(* Logix 5000 AddOnInstructionDefinition export HI1769_AOI_INT; software revision 32.00 *)

TYPE HardyCmdResult :   // Results returned for commands without specific data associated with command.
STRUCT
   Cmd : INT;
   CmdStatus : INT;
END_STRUCT
END_TYPE

TYPE HardyIntParam0 :   // parameter 0 values using integer values.
STRUCT
   ChanActive : INT;
   Metric : INT;
   Waversaver : INT;
   NumAverages : INT;
   ZeroTrackEnable : INT;
   ROC_Time_Base : INT;
   AutoZeroTol : DINT;
   MotionTol : DINT;
   ZeroTol : DINT;
   unused1 : INT;
   unused2 : INT;
END_STRUCT
END_TYPE

TYPE HardyIntParam1 :   // parameter 1 values with integer variables.
STRUCT
   TareWeight : DINT;
   SpanWeight : DINT;
   CalLowWeight : DINT;
   ZeroCount : DINT;
   CalZeroCount : DINT;
   CalLowCount : DINT;
   CalHighCount : DINT;
END_STRUCT
END_TYPE

TYPE HardyIntWeight :   // default return from module when no command given.
STRUCT
   Channel_Status : INT;
   FirmwareRev : INT;
   Gross_Weight : DINT;
   Net_Weight : DINT;
   Metric : INT;
   CalType : INT;
   ADC_Counts : DINT;
   Rate_of_Change : DINT;
   Serial_Number : INT;
   Conv_Count : INT;
END_STRUCT
END_TYPE

ADD_ON_INSTRUCTION HI1769_AOI_INT   (* revision 1.0 *)
// To operate with a single channel of an HI 1769 WS or HI 1769-2WS module.
// Revision note:
// Complete rewrite of the AOI to operate with a single channel of a module even if it is a two channel module.  This allows the user to set up each channel in the format they wish without regard to the way the other channel is configured.
VAR_IN_OUT
   Inp_hi1769 : HI:1769_xWS_ChannelNOCMD_r3:I:0; {required}
   Out_hi1769 : HI:1769_xWS_Channel:O:0; {required}
END_VAR
VAR_INPUT
   auto_zero_flt : REAL;   // auto zero tolerance float format
   auto_zero_int : DINT;   // auto zero tolerance integer format
   C2_cal_cmd : BOOL;   // trigger the C2 cal command
   cal_hi_cmd : BOOL;   // trigger the cal high command
   cal_low_cmd : BOOL;   // trigger the cal low command
   callow_wt_flt : REAL;   // Cal low reference weight float format
   callow_wt_int : DINT;   // Cal low reference weight integer format
   capacity : REAL;   // capacity of scale
   chan_enable : INT;   // Channel enabled indication
   chan_status : INT;   // channel status
   decimal_pt : INT;   // decimal point positions if integer format module
   metric : INT;   // Metric setting for units, format, decimal
   mot_tol_flt : REAL;   // motion tolerance float format
   mot_tol_int : DINT;   // motion tolerance integer format
   num_avg : INT;   // Averages
   rd_param_0_1 : BOOL;   // trigger read param 0 data from page 1 of configuration
   rd_param_0_2 : BOOL;   // trigger read param 0 data from page 2 of configuration
   rd_param_1_c2 : BOOL;   // trigger read param 1 data from C2 cal page
   rd_param_1_trad : BOOL;   // trigger read param 1 data from traditional cal page
   roc_tb : INT;   // ROC time base
   save_params0 : BOOL;   // trigger write of configuration parameters
   save_params0_2 : BOOL;   // trigger write of param0 config data from page 2 of config
   save_params1 : BOOL;   // trigger write of param 1 from C2 cal page
   save_params1_1 : BOOL;   // triggers save of cal parameters from traditional cal page
   Set_FaceplateAnimation : INT;   // sets the page of display on HMI
   span_wt_flt : REAL;   // Span ref weight float format
   span_wt_int : DINT;   // span ref weight integer format
   tare_cmd : BOOL;   // triggers tare command
   tare_wt_flt : REAL;   // tare weight float format
   tare_wt_int : DINT;   // tare weight integer format
   unit : INT;   // units of measure
   waversaver : INT;   // WAVERSAVER filter setting
   zero_cmd : BOOL;   // triggers zero command
   zero_tol_flt : REAL;   // zero tolerance float format
   zero_tol_int : DINT;   // zero tolerance integer format
   zero_trk_enable : INT;   // zero track enable
END_VAR
VAR_OUTPUT
   active : BOOL;
   cmd_status : INT;
   current_metric : INT; {access Read Only}   // current metric setting
   fp_dis_md : DINT;   // set display of gross or net weight for HMI
   gross_wt_flt : REAL; {access Read Only}   // Gross weight float format
   gross_wt_int : DINT; {access Read Only}   // gross weight integer format
   ins_status : INT;   // instrument status
   net_wt_flt : REAL; {access Read Only}   // net weight float format
   net_wt_int : DINT; {access Read Only}   // net weight integer format
   percent : REAL; {access Read Only}   // weight in percentage of capacity for gauge
   roc_flt : REAL; {access Read Only}   // Rate of Change in float format
   roc_int : DINT; {access Read Only}   // Rate of Change in integer format
END_VAR
VAR
   C2_cal_ctrl : DINT; {access None}
   C2_cmd_reset_timer : TIMER := (PRE := 3000); {access None}
   cal_data_xfer_delay : TIMER := (PRE := 200); {access None}
   cal_hi_ctrl : DINT; {access None}
   cal_lo_ctrl : DINT; {access None}
   CalHI_cmd_reset_timer : TIMER := (PRE := 3000); {access None}
   CalLo_cmd_reset_timer : TIMER := (PRE := 3000); {access None}
   clr_cmd : BOOL; {access None}
   comm_ck_timer : TIMER := (PRE := 3000); {access None}   // communications check timer
   config_data_xfer_delay_timer : TIMER := (PRE := 200); {access None}
   copy_cal_data_delay : TIMER := (PRE := 200); {access None}
   default_return_int : HardyIntWeight; {access None}
   init_metric : BOOL; {access None}
   init_timer : TIMER := (PRE := 1000); {access None}
   no_update : BOOL; {access None}   // communication loss indication
   one_shot_clr_1 : BOOL; {access None}
   one_shot_clr_2 : BOOL; {access None}
   one_shot_metric : BOOL; {access None}
   previous_count : INT; {access None}
   rd_config_data_delay : TIMER := (PRE := 200); {access None}
   rd_param0_ctrl : DINT; {access None}
   rd_param1_ctrl : DINT; {access None}
   Read_Int_param_0 : HardyIntParam0; {access None}
   Read_Int_param_1 : HardyIntParam1; {access None}
   reset_cmd_delay_timer : TIMER := (PRE := 1000); {access None}
   save_cal_delay_timer : TIMER := (PRE := 200); {access None}
   save_config_delay_timer : TIMER := (PRE := 200); {access None}
   save_param0_delay_timer : TIMER := (PRE := 3000); {access None}
   save_param1_delay_timer : TIMER := (PRE := 3000); {access None}
   start_reset_cmd_delay_timer : BOOL; {access None}   // reset read command delay
   Status_Return : HardyCmdResult; {access None}
   tare_cmd_reset_timer : TIMER := (PRE := 3000); {access None}
   tare_ctrl : DINT; {access None}
   wr_param0_ctrl : DINT; {access None}
   wr_param1_ctrl : DINT; {access None}
   write_int_param_0 : HardyIntParam0; {access None}
   write_int_param_1 : HardyIntParam1; {access None}
   zero_cmd_reset_timer : TIMER := (PRE := 3000); {access None}
   zero_ctrl : DINT; {access None}
END_VAR

ROUTINE Logic   (* ladder *)
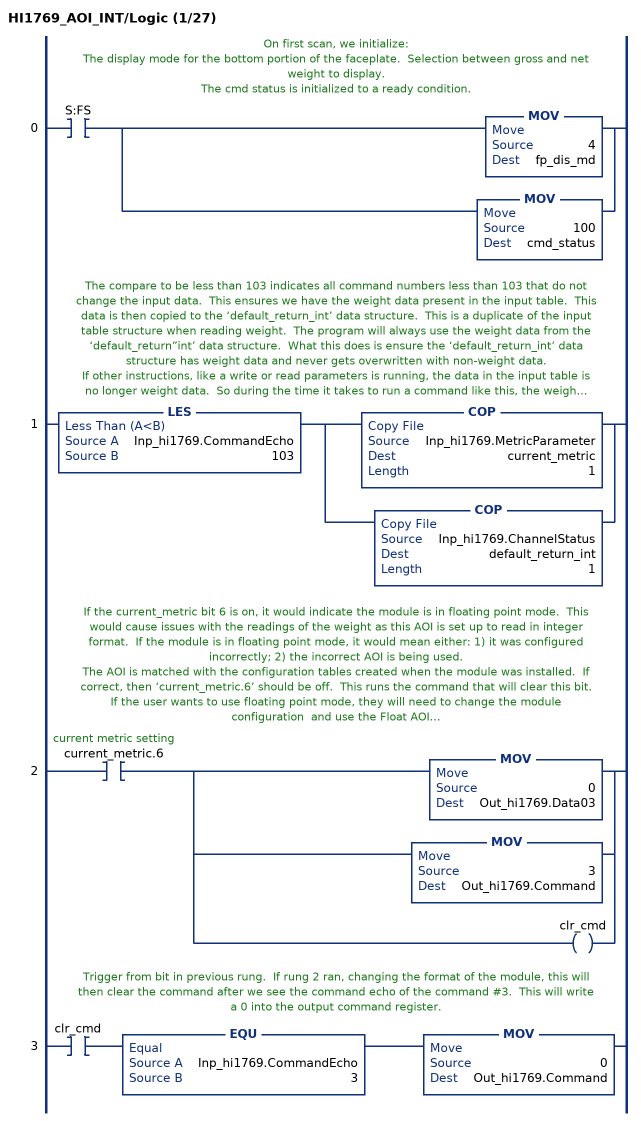
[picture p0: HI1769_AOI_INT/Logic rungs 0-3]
   // On first scan, we initialize:
   // The display mode for the bottom portion of the faceplate.  Selection between gross and net weight to display.
   // The cmd status is initialized to a ready condition.
   0: XIC(S:FS)[MOV(4,fp_dis_md) ,MOV(100,cmd_status) ];
   // The compare to be less than 103 indicates all command numbers less than 103 that do not change the input data.  This ensures we have the weight data present in the input table.  This data is then copied to the ‘default_return_int’ data structure.  This is a duplicate of the input table structure when reading weight.  The program will always use the weight data from the ‘default_return”int’ data structure.  What this does is ensure the ‘default_return_int’ data structure has weight data and never gets overwritten with non-weight data.
   // If other instructions, like a write or read parameters is running, the data in the input table is no longer weight data.  So during the time it takes to run a command like this, the weight data is taken from the ‘default_return_int’ structure instead of the input table.  The weight will not change during this time frame, but it is so short it should not matter.  However, this prevents using values as weight when the values are not weight values.
   // This also copies the metric setting to the ‘current_metric’ tag.  This tag is used to read the: Units of measure and decimal point value.
   1: LES(Inp_hi1769.CommandEcho,103)[COP(Inp_hi1769.MetricParameter,current_metric,1) ,COP(Inp_hi1769.ChannelStatus,default_return_int,1) ];
   // If the current_metric bit 6 is on, it would indicate the module is in floating point mode.  This would cause issues with the readings of the weight as this AOI is set up to read in integer format.  If the module is in floating point mode, it would mean either: 1) it was configured incorrectly; 2) the incorrect AOI is being used.
   // The AOI is matched with the configuration tables created when the module was installed.  If correct, then ‘current_metric.6’ should be off.  This runs the command that will clear this bit.
   // If the user wants to use floating point mode, they will need to change the module configuration  and use the Float AOI.
   // The command #3 writes to the metric setting in the module.  Moving the 0 into Data03 will write a 0 in for the metric setting.  This will turn off the floating point format.
   // If the bit is not set, indicating the module is in Integer format, then this rung will be skipped.
   2: XIC(current_metric.6)[MOV(0,Out_hi1769.Data03) ,MOV(3,Out_hi1769.Command) ,OTE(clr_cmd) ];
   // Trigger from bit in previous rung.  If rung 2 ran, changing the format of the module, this will then clear the command after we see the command echo of the command #3.  This will write a 0 into the output command register.
   3: XIC(clr_cmd)EQU(Inp_hi1769.CommandEcho,3)MOV(0,Out_hi1769.Command);
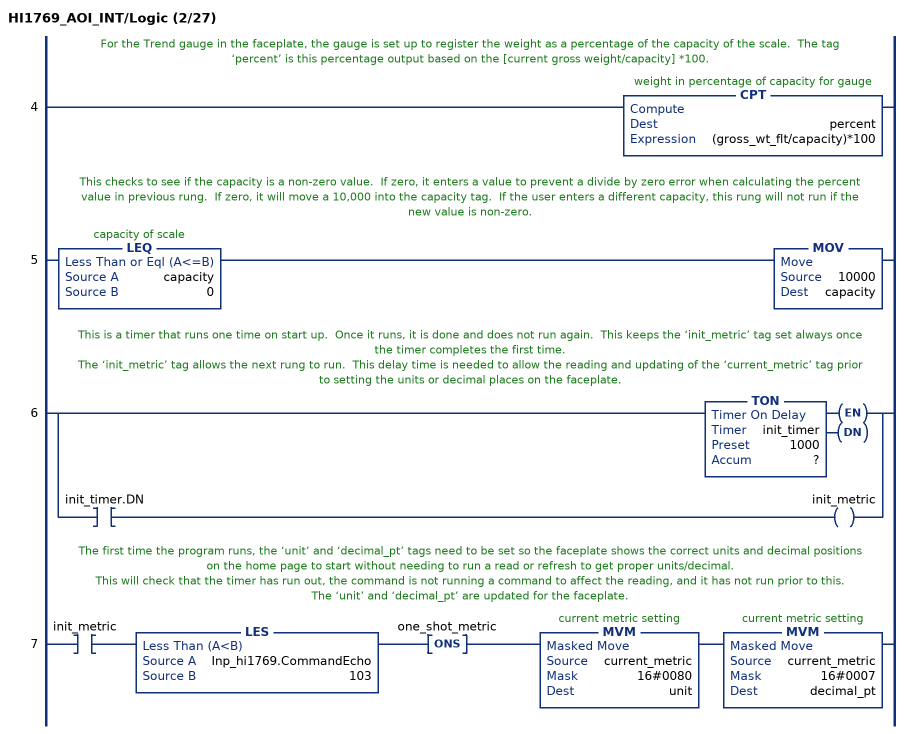
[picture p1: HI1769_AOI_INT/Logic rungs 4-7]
   // For the Trend gauge in the faceplate, the gauge is set up to register the weight as a percentage of the capacity of the scale.  The tag ‘percent’ is this percentage output based on the [current gross weight/capacity] *100.
   4: CPT(percent,(gross_wt_flt/capacity)*100);
   // This checks to see if the capacity is a non-zero value.  If zero, it enters a value to prevent a divide by zero error when calculating the percent value in previous rung.  If zero, it will move a 10,000 into the capacity tag.  If the user enters a different capacity, this rung will not run if the new value is non-zero.
   5: LEQ(capacity,0)MOV(10000,capacity);
   // This is a timer that runs one time on start up.  Once it runs, it is done and does not run again.  This keeps the ‘init_metric’ tag set always once the timer completes the first time.
   // The ‘init_metric’ tag allows the next rung to run.  This delay time is needed to allow the reading and updating of the ‘current_metric’ tag prior to setting the units or decimal places on the faceplate.
   6: [TON(init_timer,?,?) ,XIC(init_timer.DN) OTE(init_metric) ];
   // The first time the program runs, the ‘unit’ and ‘decimal_pt’ tags need to be set so the faceplate shows the correct units and decimal positions on the home page to start without needing to run a read or refresh to get proper units/decimal.
   // This will check that the timer has run out, the command is not running a command to affect the reading, and it has not run prior to this.
   // The ‘unit’ and ‘decimal_pt’ are updated for the faceplate.
   7: XIC(init_metric)LES(Inp_hi1769.CommandEcho,103)ONS(one_shot_metric)MVM(current_metric,16#0080,unit)MVM(current_metric,16#0007,decimal_pt);
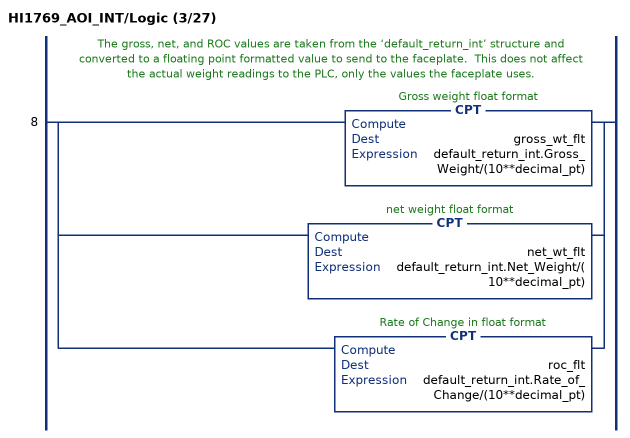
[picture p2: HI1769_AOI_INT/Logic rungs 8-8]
   // The gross, net, and ROC values are taken from the ‘default_return_int’ structure and converted to a floating point formatted value to send to the faceplate.  This does not affect the actual weight readings to the PLC, only the values the faceplate uses.
   8: [CPT(gross_wt_flt,default_return_int.Gross_Weight/(10**decimal_pt)) ,CPT(net_wt_flt,default_return_int.Net_Weight/(10**decimal_pt)) ,CPT(roc_flt,default_return_int.Rate_of_Change/(10**decimal_pt)) ];
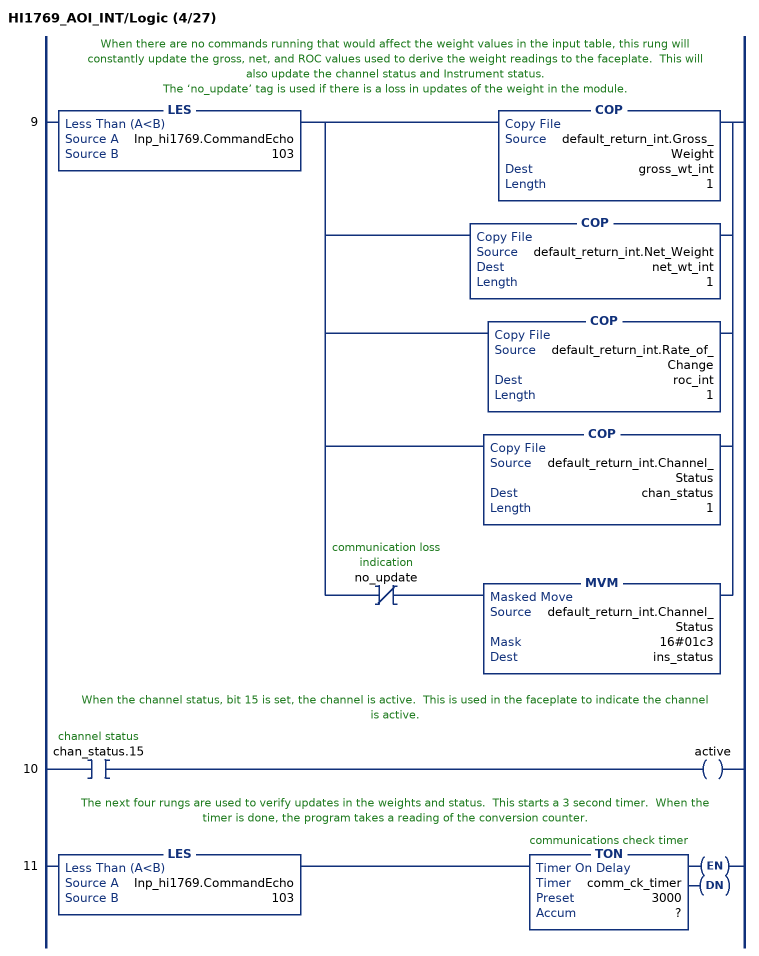
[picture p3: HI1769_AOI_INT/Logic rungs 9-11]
   // When there are no commands running that would affect the weight values in the input table, this rung will constantly update the gross, net, and ROC values used to derive the weight readings to the faceplate.  This will also update the channel status and Instrument status.
   // The ‘no_update’ tag is used if there is a loss in updates of the weight in the module.
   9: LES(Inp_hi1769.CommandEcho,103)[COP(default_return_int.Gross_Weight,gross_wt_int,1) ,COP(default_return_int.Net_Weight,net_wt_int,1) ,COP(default_return_int.Rate_of_Change,roc_int,1) ,COP(default_return_int.Channel_Status,chan_status,1) ,XIO(no_update) MVM(default_return_int.Channel_Status,16#01c3,ins_status) ];
   // When the channel status, bit 15 is set, the channel is active.  This is used in the faceplate to indicate the channel is active.
   10: XIC(chan_status.15)OTE(active);
   // The next four rungs are used to verify updates in the weights and status.  This starts a 3 second timer.  When the timer is done, the program takes a reading of the conversion counter.
   11: LES(Inp_hi1769.CommandEcho,103)TON(comm_ck_timer,?,?);
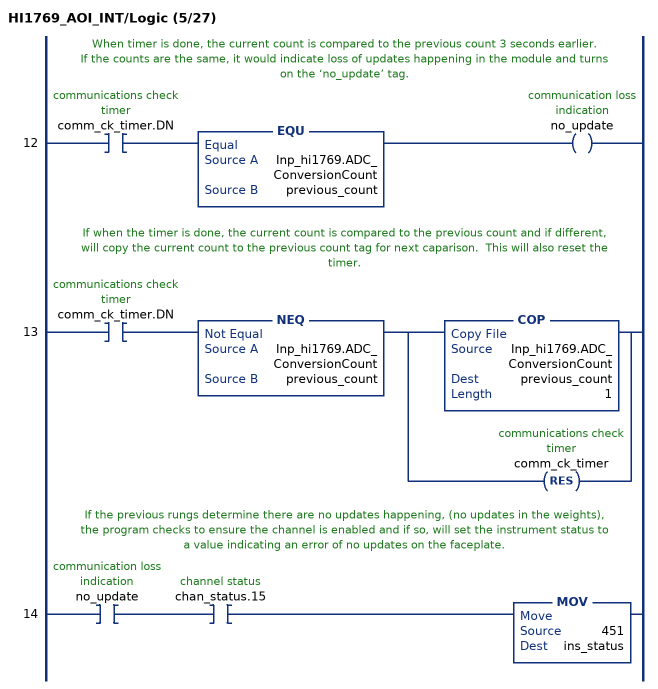
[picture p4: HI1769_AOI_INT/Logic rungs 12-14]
   // When timer is done, the current count is compared to the previous count 3 seconds earlier.
   // If the counts are the same, it would indicate loss of updates happening in the module and turns on the ‘no_update’ tag.
   12: XIC(comm_ck_timer.DN)EQU(Inp_hi1769.ADC_ConversionCount,previous_count)OTE(no_update);
   // If when the timer is done, the current count is compared to the previous count and if different, will copy the current count to the previous count tag for next caparison.  This will also reset the timer.
   13: XIC(comm_ck_timer.DN)NEQ(Inp_hi1769.ADC_ConversionCount,previous_count)[COP(Inp_hi1769.ADC_ConversionCount,previous_count,1) ,RES(comm_ck_timer) ];
   // If the previous rungs determine there are no updates happening, (no updates in the weights), the program checks to ensure the channel is enabled and if so, will set the instrument status to a value indicating an error of no updates on the faceplate.
   14: XIC(no_update)XIC(chan_status.15)MOV(451,ins_status);
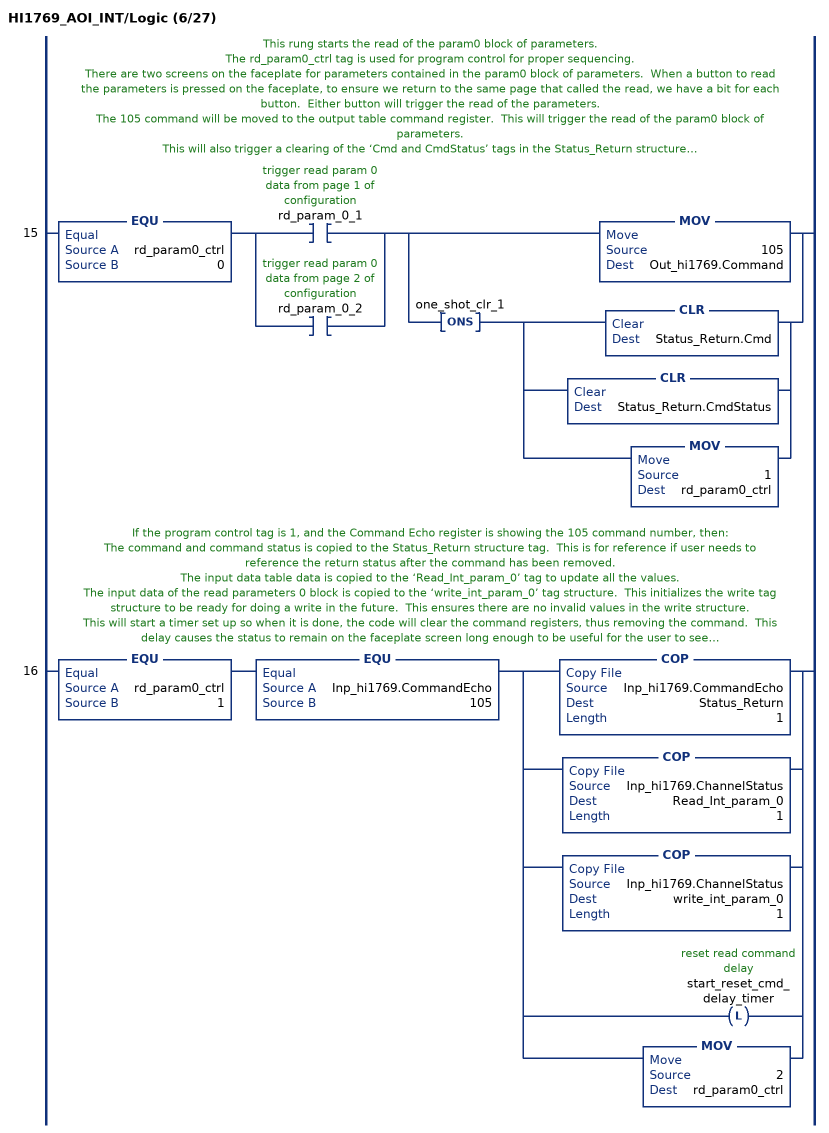
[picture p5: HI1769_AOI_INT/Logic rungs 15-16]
   // This rung starts the read of the param0 block of parameters.
   // The rd_param0_ctrl tag is used for program control for proper sequencing.
   // There are two screens on the faceplate for parameters contained in the param0 block of parameters.  When a button to read the parameters is pressed on the faceplate, to ensure we return to the same page that called the read, we have a bit for each button.  Either button will trigger the read of the parameters.
   // The 105 command will be moved to the output table command register.  This will trigger the read of the param0 block of parameters.
   // This will also trigger a clearing of the ‘Cmd and CmdStatus’ tags in the Status_Return structure.
   // The rd_param0_ctrl tag is incremented to run the next rung.
   15: EQU(rd_param0_ctrl,0)[XIC(rd_param_0_1) ,XIC(rd_param_0_2) ][MOV(105,Out_hi1769.Command) ,ONS(one_shot_clr_1) [CLR(Status_Return.Cmd) ,CLR(Status_Return.CmdStatus) ,MOV(1,rd_param0_ctrl) ] ];
   // If the program control tag is 1, and the Command Echo register is showing the 105 command number, then:
   // The command and command status is copied to the Status_Return structure tag.  This is for reference if user needs to reference the return status after the command has been removed.
   // The input data table data is copied to the ‘Read_Int_param_0’ tag to update all the values.
   // The input data of the read parameters 0 block is copied to the ‘write_int_param_0’ tag structure.  This initializes the write tag structure to be ready for doing a write in the future.  This ensures there are no invalid values in the write structure.
   // This will start a timer set up so when it is done, the code will clear the command registers, thus removing the command.  This delay causes the status to remain on the faceplate screen long enough to be useful for the user to see.
   // Increment the ctrl tag to trigger next rung.
   16: EQU(rd_param0_ctrl,1)EQU(Inp_hi1769.CommandEcho,105)[COP(Inp_hi1769.CommandEcho,Status_Return,1) ,COP(Inp_hi1769.ChannelStatus,Read_Int_param_0,1) ,COP(Inp_hi1769.ChannelStatus,write_int_param_0,1) ,OTL(start_reset_cmd_delay_timer) ,MOV(2,rd_param0_ctrl) ];
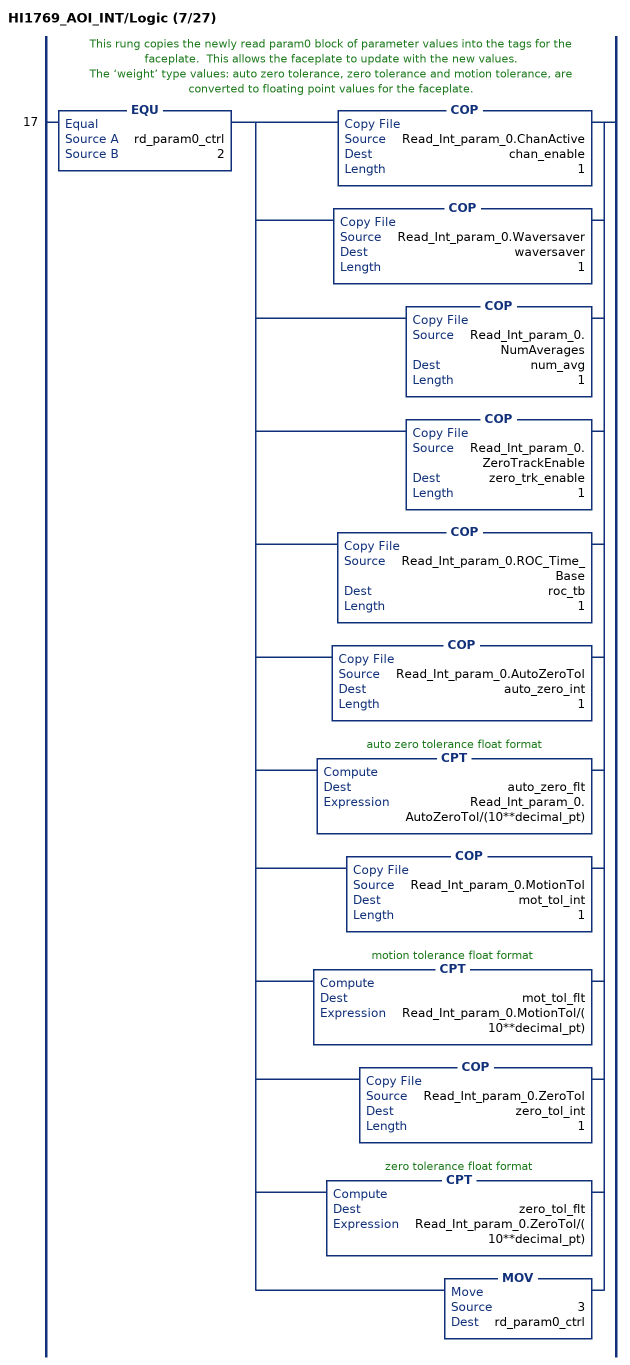
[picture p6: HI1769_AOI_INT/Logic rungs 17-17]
   // This rung copies the newly read param0 block of parameter values into the tags for the faceplate.  This allows the faceplate to update with the new values.
   // The ‘weight’ type values: auto zero tolerance, zero tolerance and motion tolerance, are converted to floating point values for the faceplate.
   17: EQU(rd_param0_ctrl,2)[COP(Read_Int_param_0.ChanActive,chan_enable,1) ,COP(Read_Int_param_0.Waversaver,waversaver,1) ,COP(Read_Int_param_0.NumAverages,num_avg,1) ,COP(Read_Int_param_0.ZeroTrackEnable,zero_trk_enable,1) ,COP(Read_Int_param_0.ROC_Time_Base,roc_tb,1) ,COP(Read_Int_param_0.AutoZeroTol,auto_zero_int,1) ,CPT(auto_zero_flt,Read_Int_param_0.AutoZeroTol/(10**decimal_pt)) ,COP(Read_Int_param_0.MotionTol,mot_tol_int,1) ,CPT(mot_tol_flt,Read_Int_param_0.MotionTol/(10**decimal_pt)) ,COP(Read_Int_param_0.ZeroTol,zero_tol_int,1) ,CPT(zero_tol_flt,Read_Int_param_0.ZeroTol/(10**decimal_pt)) ,MOV(3,rd_param0_ctrl) ];
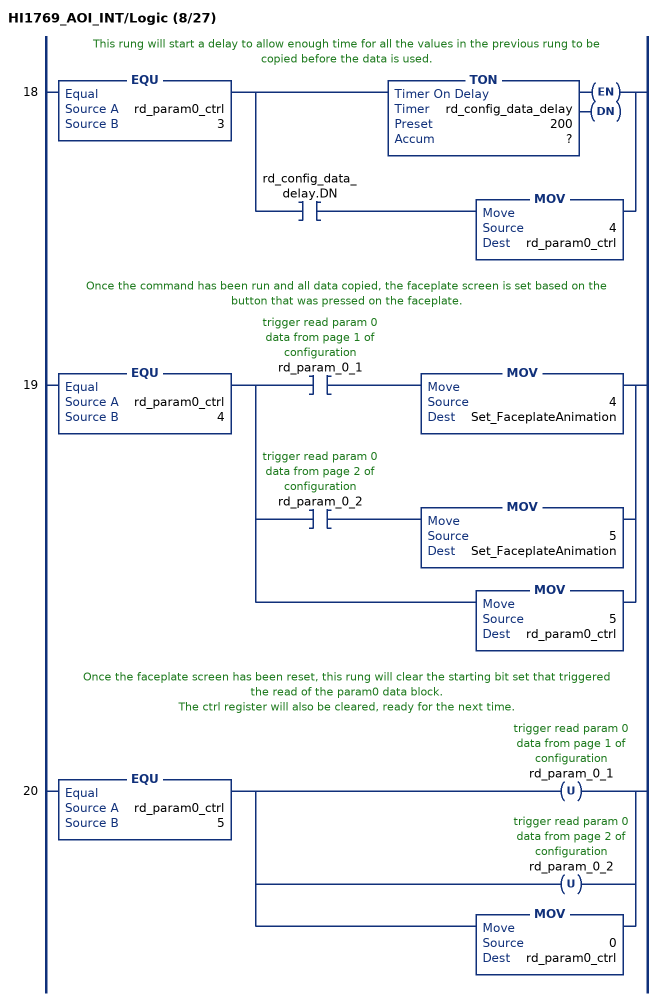
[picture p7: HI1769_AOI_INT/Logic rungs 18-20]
   // This rung will start a delay to allow enough time for all the values in the previous rung to be copied before the data is used.
   18: EQU(rd_param0_ctrl,3)[TON(rd_config_data_delay,?,?) ,XIC(rd_config_data_delay.DN) MOV(4,rd_param0_ctrl) ];
   // Once the command has been run and all data copied, the faceplate screen is set based on the button that was pressed on the faceplate.
   19: EQU(rd_param0_ctrl,4)[XIC(rd_param_0_1) MOV(4,Set_FaceplateAnimation) ,XIC(rd_param_0_2) MOV(5,Set_FaceplateAnimation) ,MOV(5,rd_param0_ctrl) ];
   // Once the faceplate screen has been reset, this rung will clear the starting bit set that triggered the read of the param0 data block.
   // The ctrl register will also be cleared, ready for the next time.
   20: EQU(rd_param0_ctrl,5)[OTU(rd_param_0_1) ,OTU(rd_param_0_2) ,MOV(0,rd_param0_ctrl) ];
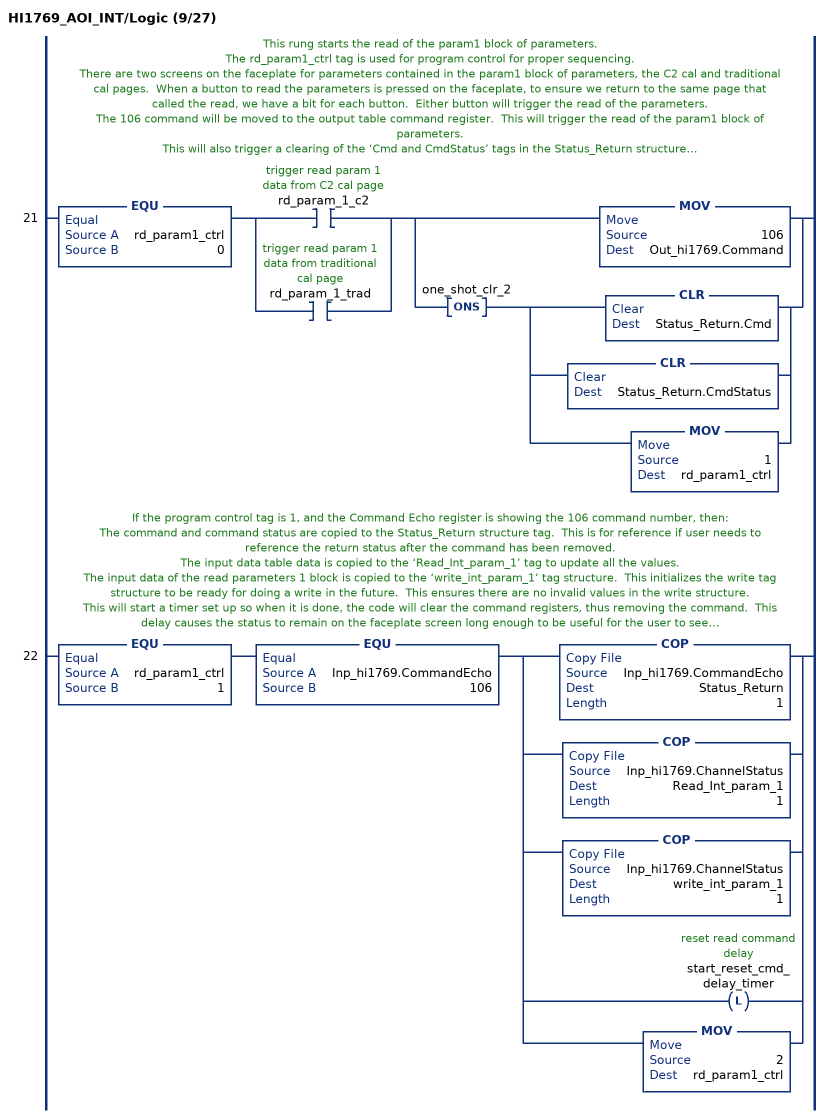
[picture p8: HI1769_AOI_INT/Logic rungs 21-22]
   // This rung starts the read of the param1 block of parameters.
   // The rd_param1_ctrl tag is used for program control for proper sequencing.
   // There are two screens on the faceplate for parameters contained in the param1 block of parameters, the C2 cal and traditional cal pages.  When a button to read the parameters is pressed on the faceplate, to ensure we return to the same page that called the read, we have a bit for each button.  Either button will trigger the read of the parameters.
   // The 106 command will be moved to the output table command register.  This will trigger the read of the param1 block of parameters.
   // This will also trigger a clearing of the ‘Cmd and CmdStatus’ tags in the Status_Return structure.
   // The rd_param1_ctrl tag is incremented to run the next rung.
   21: EQU(rd_param1_ctrl,0)[XIC(rd_param_1_c2) ,XIC(rd_param_1_trad) ][MOV(106,Out_hi1769.Command) ,ONS(one_shot_clr_2) [CLR(Status_Return.Cmd) ,CLR(Status_Return.CmdStatus) ,MOV(1,rd_param1_ctrl) ] ];
   // If the program control tag is 1, and the Command Echo register is showing the 106 command number, then:
   // The command and command status are copied to the Status_Return structure tag.  This is for reference if user needs to reference the return status after the command has been removed.
   // The input data table data is copied to the ‘Read_Int_param_1’ tag to update all the values.
   // The input data of the read parameters 1 block is copied to the ‘write_int_param_1’ tag structure.  This initializes the write tag structure to be ready for doing a write in the future.  This ensures there are no invalid values in the write structure.
   // This will start a timer set up so when it is done, the code will clear the command registers, thus removing the command.  This delay causes the status to remain on the faceplate screen long enough to be useful for the user to see.
   // Increment the ctrl tag to trigger next rung.
   22: EQU(rd_param1_ctrl,1)EQU(Inp_hi1769.CommandEcho,106)[COP(Inp_hi1769.CommandEcho,Status_Return,1) ,COP(Inp_hi1769.ChannelStatus,Read_Int_param_1,1) ,COP(Inp_hi1769.ChannelStatus,write_int_param_1,1) ,OTL(start_reset_cmd_delay_timer) ,MOV(2,rd_param1_ctrl) ];
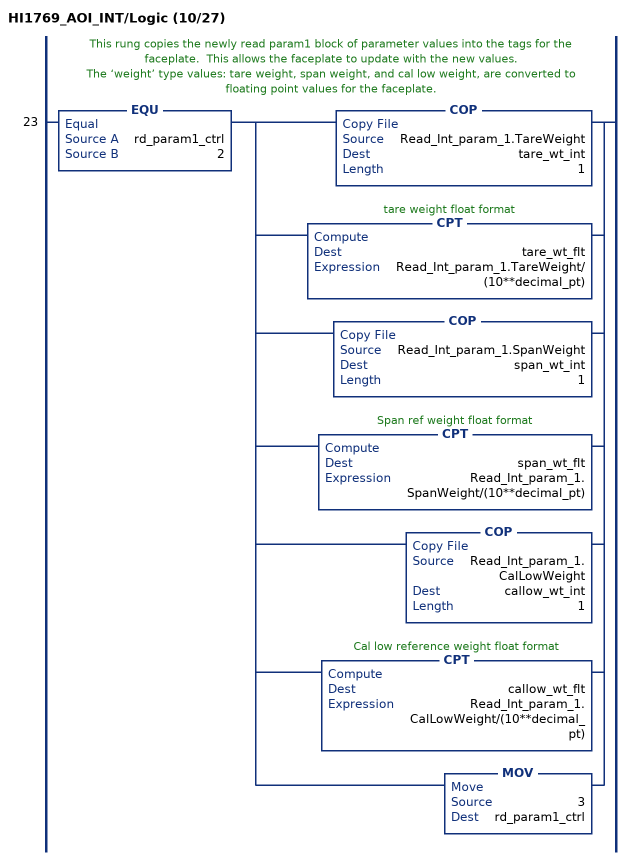
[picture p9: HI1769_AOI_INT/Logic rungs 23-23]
   // This rung copies the newly read param1 block of parameter values into the tags for the faceplate.  This allows the faceplate to update with the new values.
   // The ‘weight’ type values: tare weight, span weight, and cal low weight, are converted to floating point values for the faceplate.
   23: EQU(rd_param1_ctrl,2)[COP(Read_Int_param_1.TareWeight,tare_wt_int,1) ,CPT(tare_wt_flt,Read_Int_param_1.TareWeight/(10**decimal_pt)) ,COP(Read_Int_param_1.SpanWeight,span_wt_int,1) ,CPT(span_wt_flt,Read_Int_param_1.SpanWeight/(10**decimal_pt)) ,COP(Read_Int_param_1.CalLowWeight,callow_wt_int,1) ,CPT(callow_wt_flt,Read_Int_param_1.CalLowWeight/(10**decimal_pt)) ,MOV(3,rd_param1_ctrl) ];
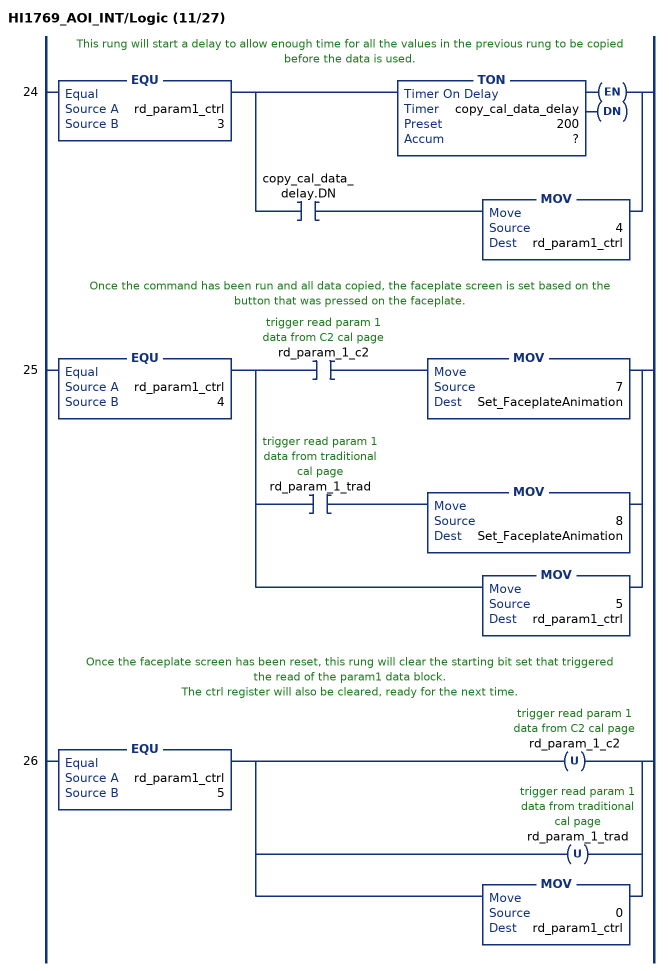
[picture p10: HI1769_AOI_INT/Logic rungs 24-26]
   // This rung will start a delay to allow enough time for all the values in the previous rung to be copied before the data is used.
   24: EQU(rd_param1_ctrl,3)[TON(copy_cal_data_delay,?,?) ,XIC(copy_cal_data_delay.DN) MOV(4,rd_param1_ctrl) ];
   // Once the command has been run and all data copied, the faceplate screen is set based on the button that was pressed on the faceplate.
   25: EQU(rd_param1_ctrl,4)[XIC(rd_param_1_c2) MOV(7,Set_FaceplateAnimation) ,XIC(rd_param_1_trad) MOV(8,Set_FaceplateAnimation) ,MOV(5,rd_param1_ctrl) ];
   // Once the faceplate screen has been reset, this rung will clear the starting bit set that triggered the read of the param1 data block.
   // The ctrl register will also be cleared, ready for the next time.
   26: EQU(rd_param1_ctrl,5)[OTU(rd_param_1_c2) ,OTU(rd_param_1_trad) ,MOV(0,rd_param1_ctrl) ];
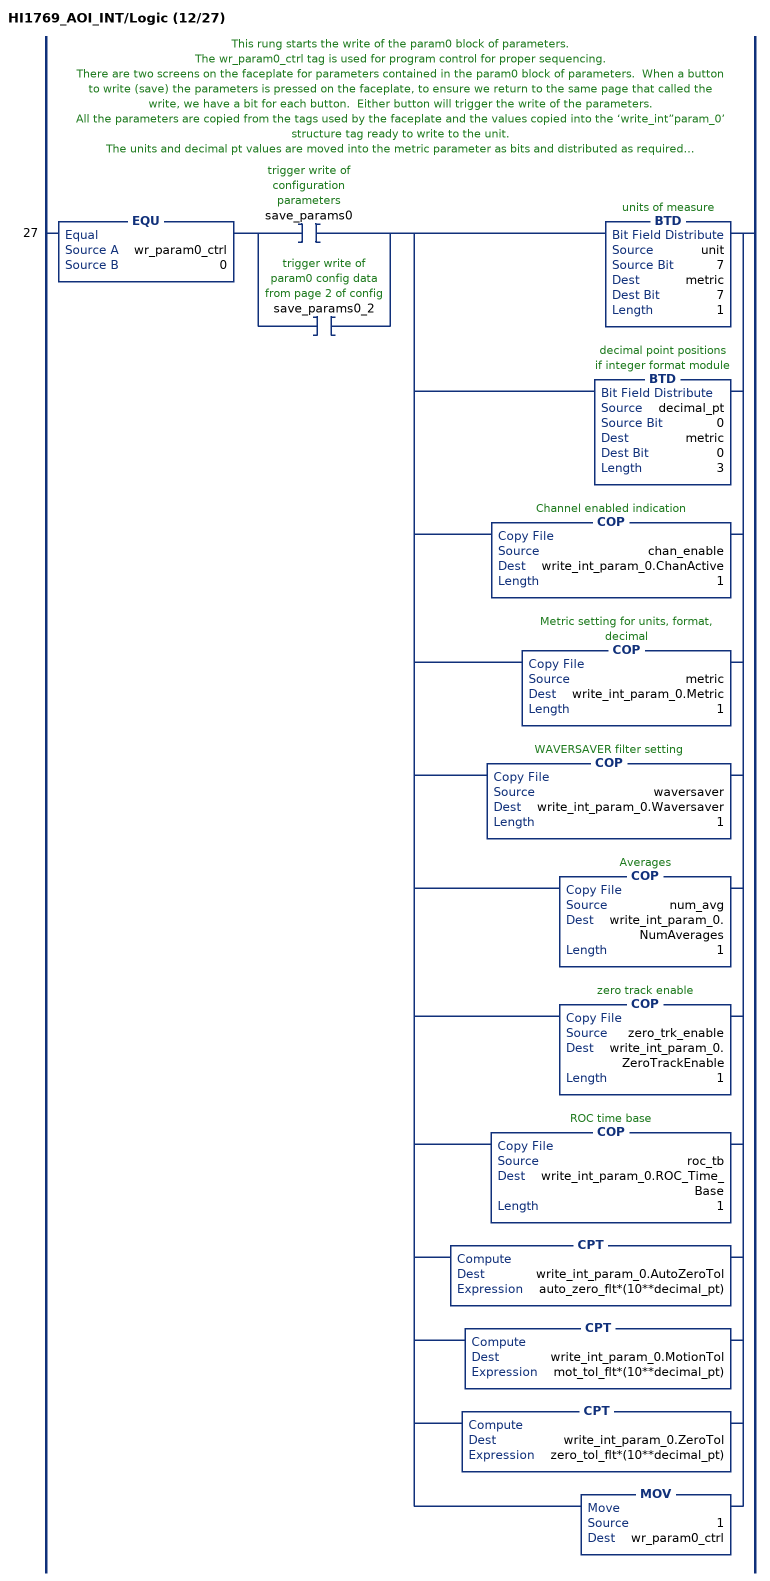
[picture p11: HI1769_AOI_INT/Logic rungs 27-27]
   // This rung starts the write of the param0 block of parameters.
   // The wr_param0_ctrl tag is used for program control for proper sequencing.
   // There are two screens on the faceplate for parameters contained in the param0 block of parameters.  When a button to write (save) the parameters is pressed on the faceplate, to ensure we return to the same page that called the write, we have a bit for each button.  Either button will trigger the write of the parameters.
   // All the parameters are copied from the tags used by the faceplate and the values copied into the ‘write_int”param_0’ structure tag ready to write to the unit.
   // The units and decimal pt values are moved into the metric parameter as bits and distributed as required.
   // The weight type values, auto zero tolerance, motion tolerance, and zero tolerance, are converted to integer data type with the proper resolution based on the decimal pt tag setting.
   27: EQU(wr_param0_ctrl,0)[XIC(save_params0) ,XIC(save_params0_2) ][BTD(unit,7,metric,7,1) ,BTD(decimal_pt,0,metric,0,3) ,COP(chan_enable,write_int_param_0.ChanActive,1) ,COP(metric,write_int_param_0.Metric,1) ,COP(waversaver,write_int_param_0.Waversaver,1) ,COP(num_avg,write_int_param_0.NumAverages,1) ,COP(zero_trk_enable,write_int_param_0.ZeroTrackEnable,1) ,COP(roc_tb,write_int_param_0.ROC_Time_Base,1) ,CPT(write_int_param_0.AutoZeroTol,auto_zero_flt*(10**decimal_pt)) ,CPT(write_int_param_0.MotionTol,mot_tol_flt*(10**decimal_pt)) ,CPT(write_int_param_0.ZeroTol,zero_tol_flt*(10**decimal_pt)) ,MOV(1,wr_param0_ctrl) ];
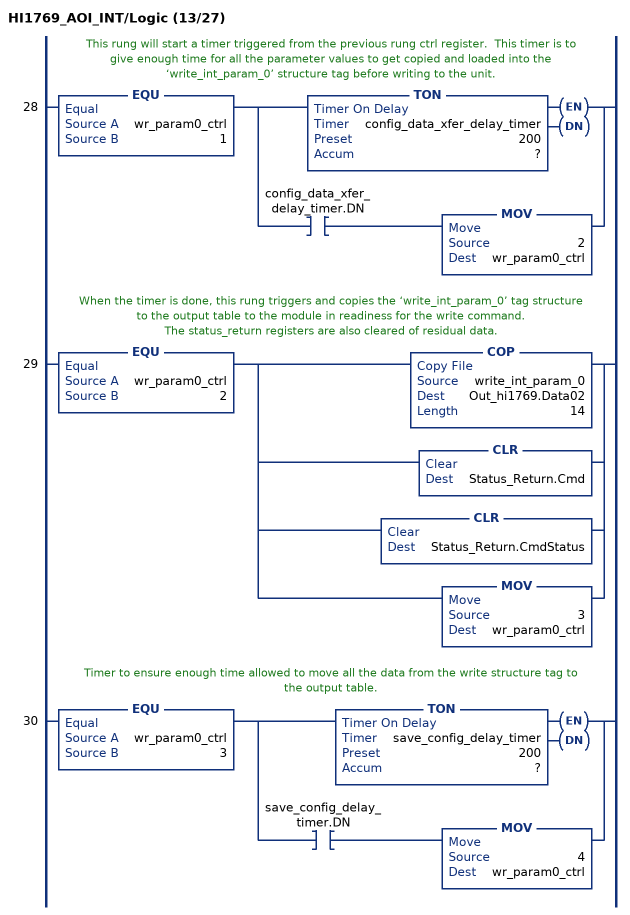
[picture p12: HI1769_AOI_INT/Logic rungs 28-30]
   // This rung will start a timer triggered from the previous rung ctrl register.  This timer is to give enough time for all the parameter values to get copied and loaded into the ‘write_int_param_0’ structure tag before writing to the unit.
   28: EQU(wr_param0_ctrl,1)[TON(config_data_xfer_delay_timer,?,?) ,XIC(config_data_xfer_delay_timer.DN) MOV(2,wr_param0_ctrl) ];
   // When the timer is done, this rung triggers and copies the ‘write_int_param_0’ tag structure to the output table to the module in readiness for the write command.
   // The status_return registers are also cleared of residual data.
   29: EQU(wr_param0_ctrl,2)[COP(write_int_param_0,Out_hi1769.Data02,14) ,CLR(Status_Return.Cmd) ,CLR(Status_Return.CmdStatus) ,MOV(3,wr_param0_ctrl) ];
   // Timer to ensure enough time allowed to move all the data from the write structure tag to the output table.
   30: EQU(wr_param0_ctrl,3)[TON(save_config_delay_timer,?,?) ,XIC(save_config_delay_timer.DN) MOV(4,wr_param0_ctrl) ];
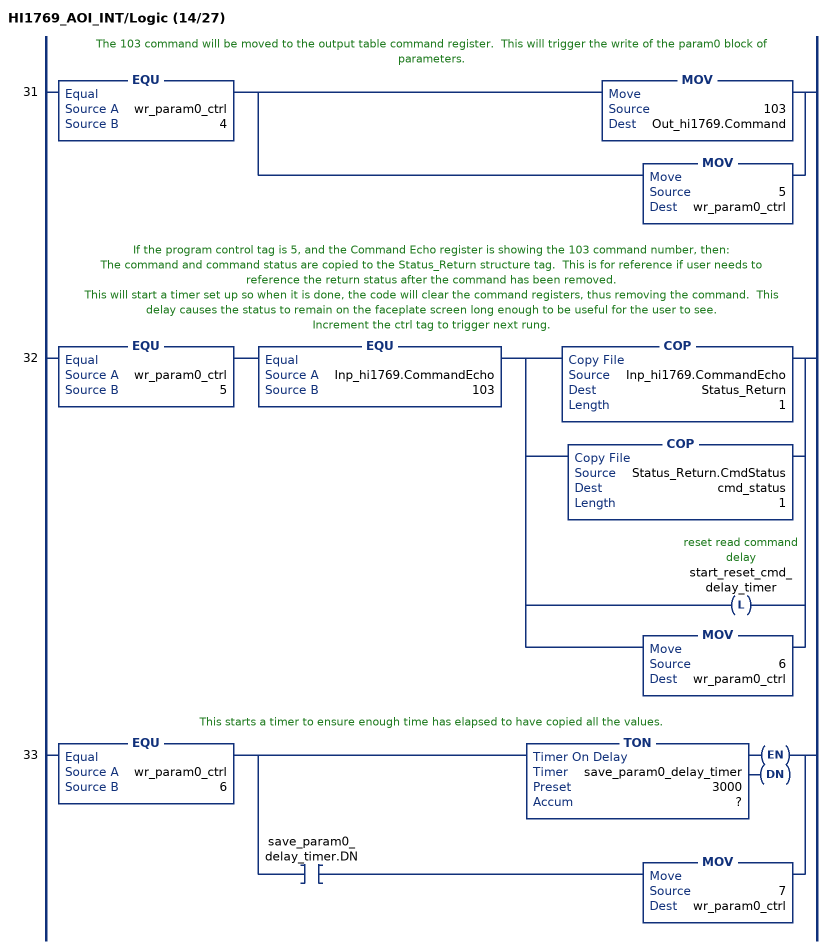
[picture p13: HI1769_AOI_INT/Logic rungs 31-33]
   // The 103 command will be moved to the output table command register.  This will trigger the write of the param0 block of parameters.
   31: EQU(wr_param0_ctrl,4)[MOV(103,Out_hi1769.Command) ,MOV(5,wr_param0_ctrl) ];
   // If the program control tag is 5, and the Command Echo register is showing the 103 command number, then:
   // The command and command status are copied to the Status_Return structure tag.  This is for reference if user needs to reference the return status after the command has been removed.
   // This will start a timer set up so when it is done, the code will clear the command registers, thus removing the command.  This delay causes the status to remain on the faceplate screen long enough to be useful for the user to see.
   // Increment the ctrl tag to trigger next rung.
   32: EQU(wr_param0_ctrl,5)EQU(Inp_hi1769.CommandEcho,103)[COP(Inp_hi1769.CommandEcho,Status_Return,1) ,COP(Status_Return.CmdStatus,cmd_status,1) ,OTL(start_reset_cmd_delay_timer) ,MOV(6,wr_param0_ctrl) ];
   // This starts a timer to ensure enough time has elapsed to have copied all the values.
   33: EQU(wr_param0_ctrl,6)[TON(save_param0_delay_timer,?,?) ,XIC(save_param0_delay_timer.DN) MOV(7,wr_param0_ctrl) ];
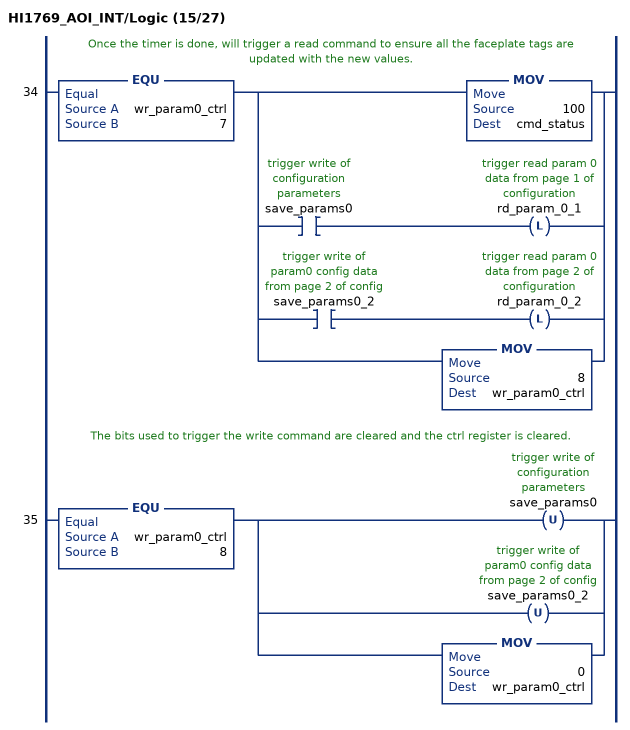
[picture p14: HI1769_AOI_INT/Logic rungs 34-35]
   // Once the timer is done, will trigger a read command to ensure all the faceplate tags are updated with the new values.
   34: EQU(wr_param0_ctrl,7)[MOV(100,cmd_status) ,XIC(save_params0) OTL(rd_param_0_1) ,XIC(save_params0_2) OTL(rd_param_0_2) ,MOV(8,wr_param0_ctrl) ];
   // The bits used to trigger the write command are cleared and the ctrl register is cleared.
   35: EQU(wr_param0_ctrl,8)[OTU(save_params0) ,OTU(save_params0_2) ,MOV(0,wr_param0_ctrl) ];
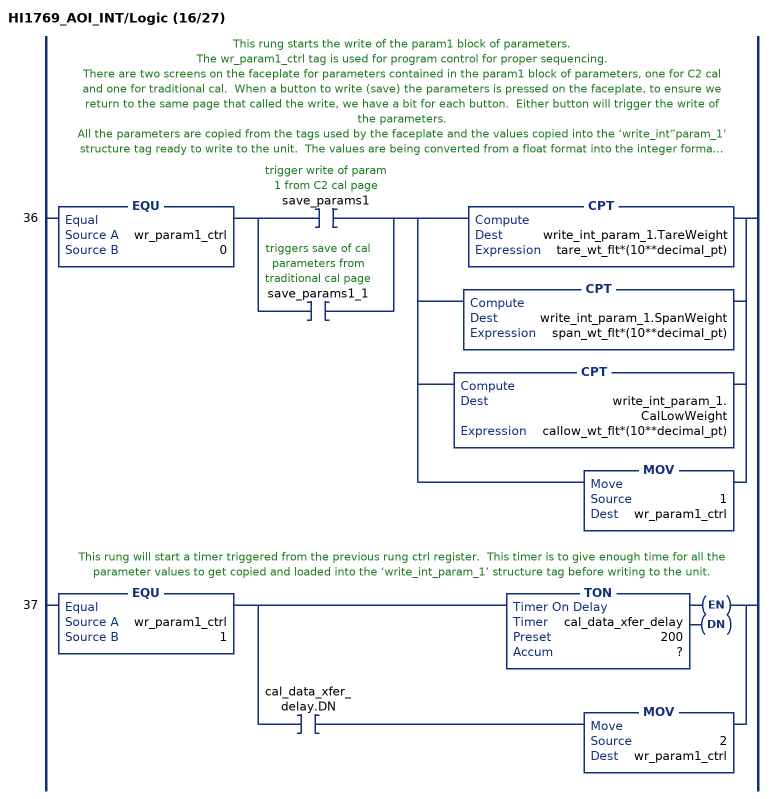
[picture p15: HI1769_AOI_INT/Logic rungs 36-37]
   // This rung starts the write of the param1 block of parameters.
   // The wr_param1_ctrl tag is used for program control for proper sequencing.
   // There are two screens on the faceplate for parameters contained in the param1 block of parameters, one for C2 cal and one for traditional cal.  When a button to write (save) the parameters is pressed on the faceplate, to ensure we return to the same page that called the write, we have a bit for each button.  Either button will trigger the write of the parameters.
   // All the parameters are copied from the tags used by the faceplate and the values copied into the ‘write_int”param_1’ structure tag ready to write to the unit.  The values are being converted from a float format into the integer format with proper decimal resolution.
   36: EQU(wr_param1_ctrl,0)[XIC(save_params1) ,XIC(save_params1_1) ][CPT(write_int_param_1.TareWeight,tare_wt_flt*(10**decimal_pt)) ,CPT(write_int_param_1.SpanWeight,span_wt_flt*(10**decimal_pt)) ,CPT(write_int_param_1.CalLowWeight,callow_wt_flt*(10**decimal_pt)) ,MOV(1,wr_param1_ctrl) ];
   // This rung will start a timer triggered from the previous rung ctrl register.  This timer is to give enough time for all the parameter values to get copied and loaded into the ‘write_int_param_1’ structure tag before writing to the unit.
   37: EQU(wr_param1_ctrl,1)[TON(cal_data_xfer_delay,?,?) ,XIC(cal_data_xfer_delay.DN) MOV(2,wr_param1_ctrl) ];
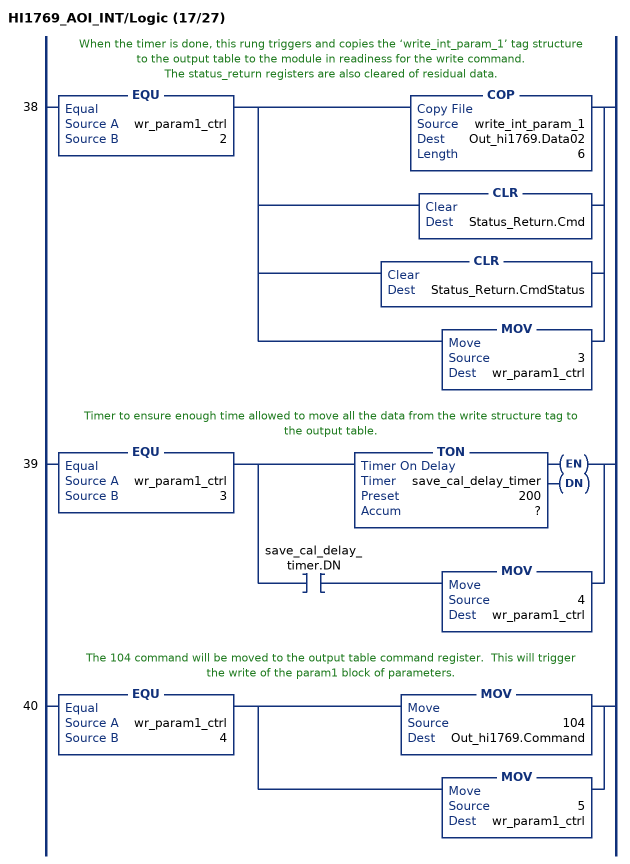
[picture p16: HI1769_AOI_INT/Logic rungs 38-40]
   // When the timer is done, this rung triggers and copies the ‘write_int_param_1’ tag structure to the output table to the module in readiness for the write command.
   // The status_return registers are also cleared of residual data.
   38: EQU(wr_param1_ctrl,2)[COP(write_int_param_1,Out_hi1769.Data02,6) ,CLR(Status_Return.Cmd) ,CLR(Status_Return.CmdStatus) ,MOV(3,wr_param1_ctrl) ];
   // Timer to ensure enough time allowed to move all the data from the write structure tag to the output table.
   39: EQU(wr_param1_ctrl,3)[TON(save_cal_delay_timer,?,?) ,XIC(save_cal_delay_timer.DN) MOV(4,wr_param1_ctrl) ];
   // The 104 command will be moved to the output table command register.  This will trigger the write of the param1 block of parameters.
   40: EQU(wr_param1_ctrl,4)[MOV(104,Out_hi1769.Command) ,MOV(5,wr_param1_ctrl) ];
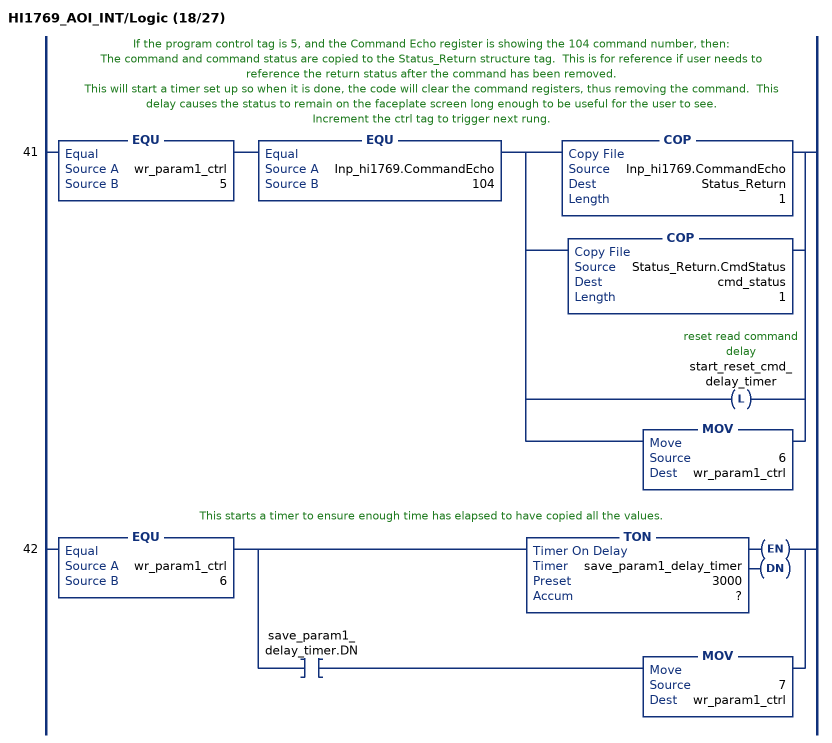
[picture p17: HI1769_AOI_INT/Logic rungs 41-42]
   // If the program control tag is 5, and the Command Echo register is showing the 104 command number, then:
   // The command and command status are copied to the Status_Return structure tag.  This is for reference if user needs to reference the return status after the command has been removed.
   // This will start a timer set up so when it is done, the code will clear the command registers, thus removing the command.  This delay causes the status to remain on the faceplate screen long enough to be useful for the user to see.
   // Increment the ctrl tag to trigger next rung.
   41: EQU(wr_param1_ctrl,5)EQU(Inp_hi1769.CommandEcho,104)[COP(Inp_hi1769.CommandEcho,Status_Return,1) ,COP(Status_Return.CmdStatus,cmd_status,1) ,OTL(start_reset_cmd_delay_timer) ,MOV(6,wr_param1_ctrl) ];
   // This starts a timer to ensure enough time has elapsed to have copied all the values.
   42: EQU(wr_param1_ctrl,6)[TON(save_param1_delay_timer,?,?) ,XIC(save_param1_delay_timer.DN) MOV(7,wr_param1_ctrl) ];
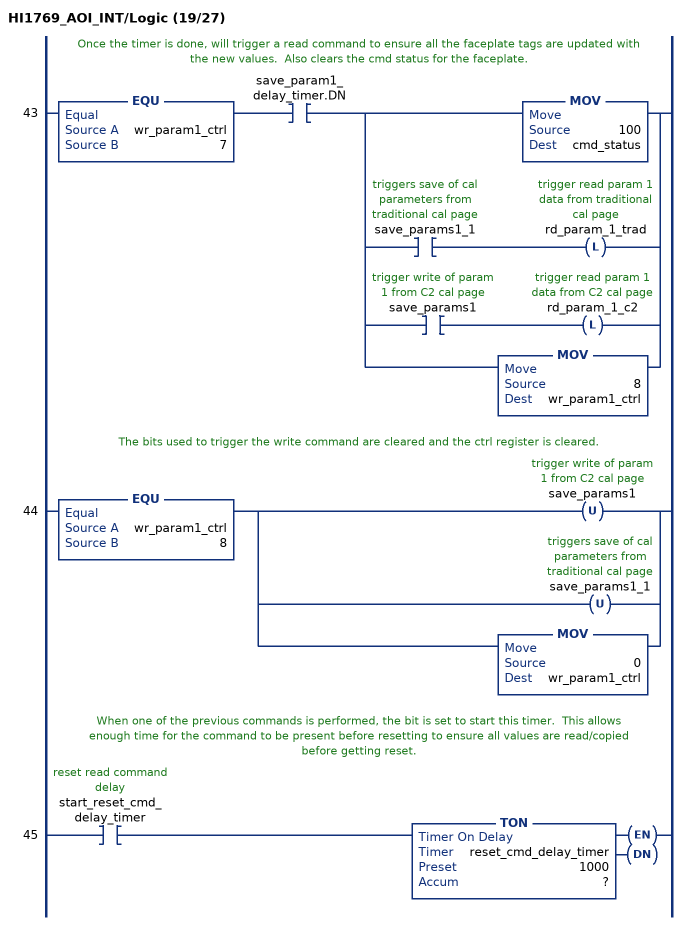
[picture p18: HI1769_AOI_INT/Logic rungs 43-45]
   // Once the timer is done, will trigger a read command to ensure all the faceplate tags are updated with the new values.  Also clears the cmd status for the faceplate.
   43: EQU(wr_param1_ctrl,7)XIC(save_param1_delay_timer.DN)[MOV(100,cmd_status) ,XIC(save_params1_1) OTL(rd_param_1_trad) ,XIC(save_params1) OTL(rd_param_1_c2) ,MOV(8,wr_param1_ctrl) ];
   // The bits used to trigger the write command are cleared and the ctrl register is cleared.
   44: EQU(wr_param1_ctrl,8)[OTU(save_params1) ,OTU(save_params1_1) ,MOV(0,wr_param1_ctrl) ];
   // When one of the previous commands is performed, the bit is set to start this timer.  This allows enough time for the command to be present before resetting to ensure all values are read/copied before getting reset.
   45: XIC(start_reset_cmd_delay_timer)TON(reset_cmd_delay_timer,?,?);
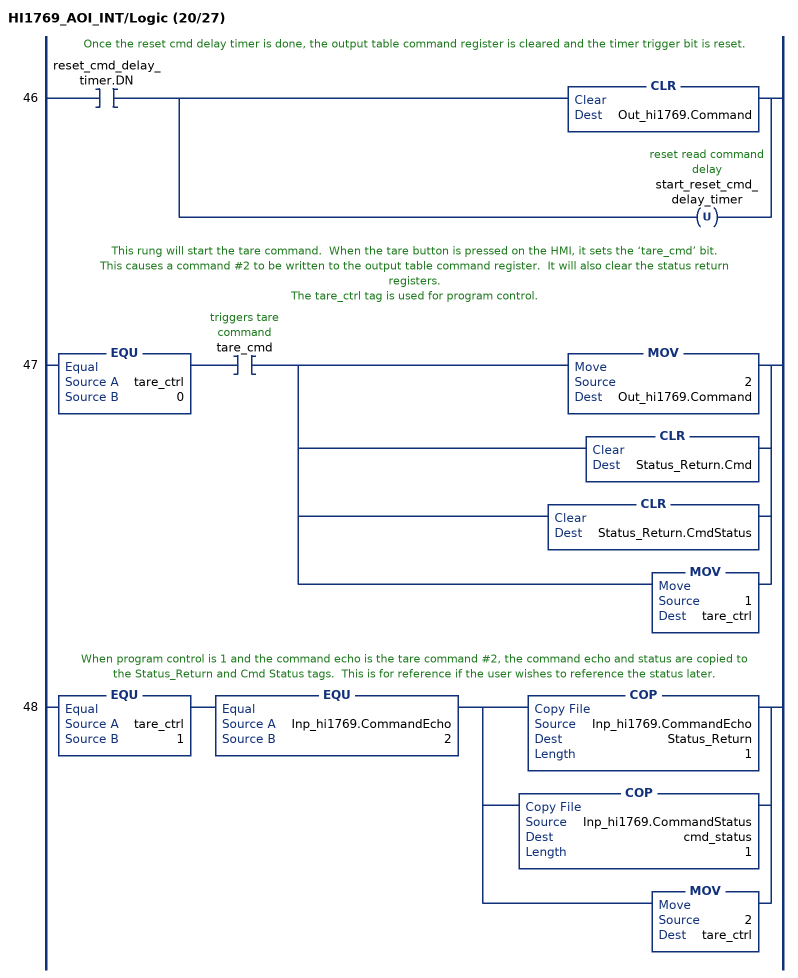
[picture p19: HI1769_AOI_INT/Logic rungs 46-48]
   // Once the reset cmd delay timer is done, the output table command register is cleared and the timer trigger bit is reset.
   46: XIC(reset_cmd_delay_timer.DN)[CLR(Out_hi1769.Command) ,OTU(start_reset_cmd_delay_timer) ];
   // This rung will start the tare command.  When the tare button is pressed on the HMI, it sets the ‘tare_cmd’ bit.
   // This causes a command #2 to be written to the output table command register.  It will also clear the status return registers.
   // The tare_ctrl tag is used for program control.
   47: EQU(tare_ctrl,0)XIC(tare_cmd)[MOV(2,Out_hi1769.Command) ,CLR(Status_Return.Cmd) ,CLR(Status_Return.CmdStatus) ,MOV(1,tare_ctrl) ];
   // When program control is 1 and the command echo is the tare command #2, the command echo and status are copied to the Status_Return and Cmd Status tags.  This is for reference if the user wishes to reference the status later.
   48: EQU(tare_ctrl,1)EQU(Inp_hi1769.CommandEcho,2)[COP(Inp_hi1769.CommandEcho,Status_Return,1) ,COP(Inp_hi1769.CommandStatus,cmd_status,1) ,MOV(2,tare_ctrl) ];
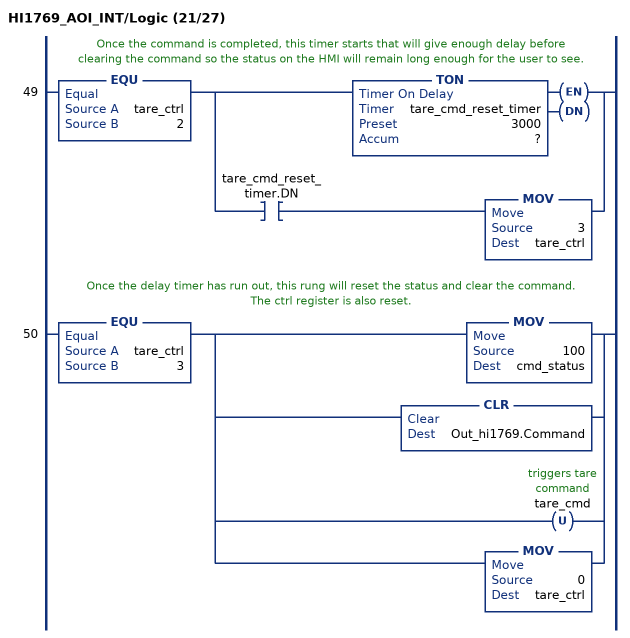
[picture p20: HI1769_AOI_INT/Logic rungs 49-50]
   // Once the command is completed, this timer starts that will give enough delay before clearing the command so the status on the HMI will remain long enough for the user to see.
   49: EQU(tare_ctrl,2)[TON(tare_cmd_reset_timer,?,?) ,XIC(tare_cmd_reset_timer.DN) MOV(3,tare_ctrl) ];
   // Once the delay timer has run out, this rung will reset the status and clear the command.
   // The ctrl register is also reset.
   50: EQU(tare_ctrl,3)[MOV(100,cmd_status) ,CLR(Out_hi1769.Command) ,OTU(tare_cmd) ,MOV(0,tare_ctrl) ];
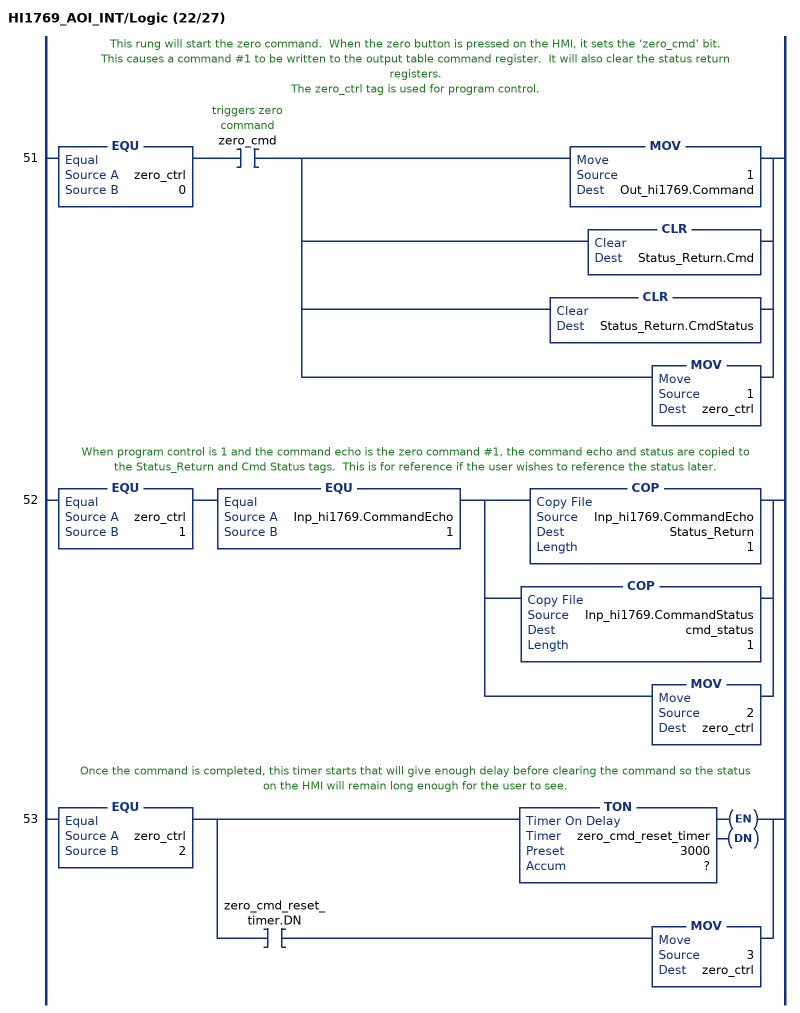
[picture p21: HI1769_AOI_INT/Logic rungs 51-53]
   // This rung will start the zero command.  When the zero button is pressed on the HMI, it sets the ‘zero_cmd’ bit.
   // This causes a command #1 to be written to the output table command register.  It will also clear the status return registers.
   // The zero_ctrl tag is used for program control.
   51: EQU(zero_ctrl,0)XIC(zero_cmd)[MOV(1,Out_hi1769.Command) ,CLR(Status_Return.Cmd) ,CLR(Status_Return.CmdStatus) ,MOV(1,zero_ctrl) ];
   // When program control is 1 and the command echo is the zero command #1, the command echo and status are copied to the Status_Return and Cmd Status tags.  This is for reference if the user wishes to reference the status later.
   52: EQU(zero_ctrl,1)EQU(Inp_hi1769.CommandEcho,1)[COP(Inp_hi1769.CommandEcho,Status_Return,1) ,COP(Inp_hi1769.CommandStatus,cmd_status,1) ,MOV(2,zero_ctrl) ];
   // Once the command is completed, this timer starts that will give enough delay before clearing the command so the status on the HMI will remain long enough for the user to see.
   53: EQU(zero_ctrl,2)[TON(zero_cmd_reset_timer,?,?) ,XIC(zero_cmd_reset_timer.DN) MOV(3,zero_ctrl) ];
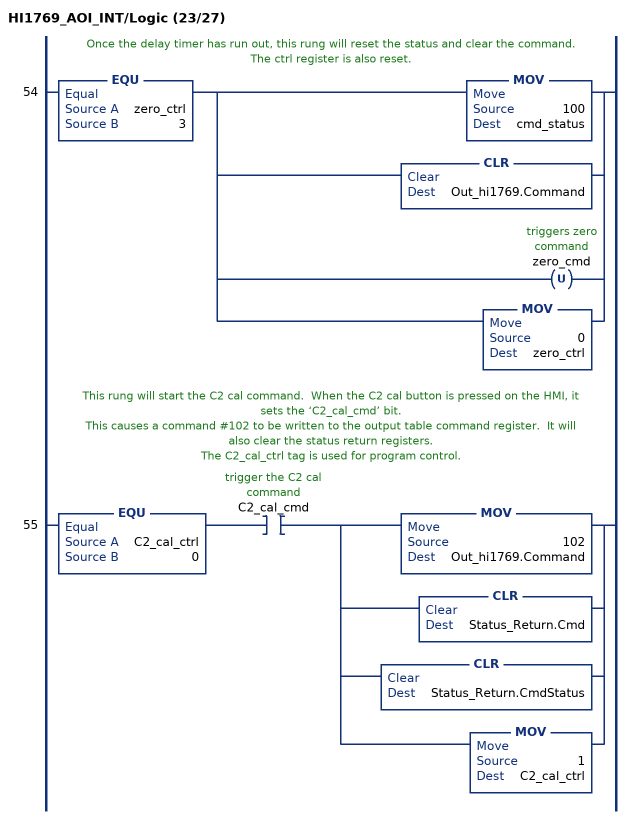
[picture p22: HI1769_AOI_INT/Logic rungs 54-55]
   // Once the delay timer has run out, this rung will reset the status and clear the command.
   // The ctrl register is also reset.
   54: EQU(zero_ctrl,3)[MOV(100,cmd_status) ,CLR(Out_hi1769.Command) ,OTU(zero_cmd) ,MOV(0,zero_ctrl) ];
   // This rung will start the C2 cal command.  When the C2 cal button is pressed on the HMI, it sets the ‘C2_cal_cmd’ bit.
   // This causes a command #102 to be written to the output table command register.  It will also clear the status return registers.
   // The C2_cal_ctrl tag is used for program control.
   55: EQU(C2_cal_ctrl,0)XIC(C2_cal_cmd)[MOV(102,Out_hi1769.Command) ,CLR(Status_Return.Cmd) ,CLR(Status_Return.CmdStatus) ,MOV(1,C2_cal_ctrl) ];
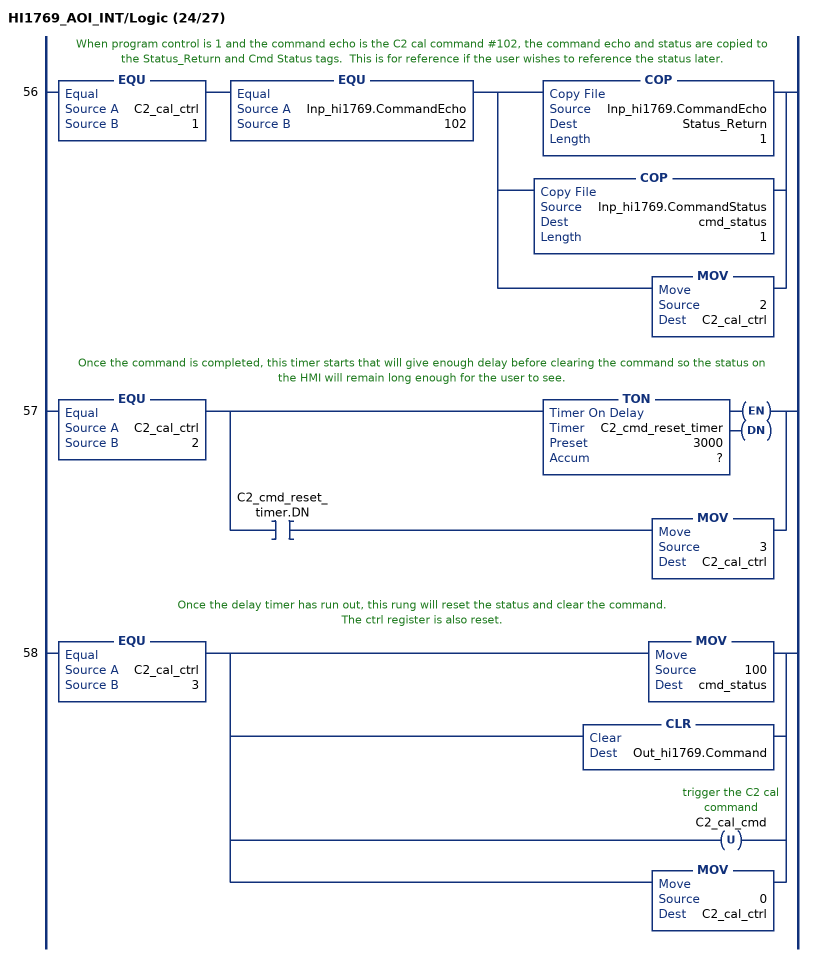
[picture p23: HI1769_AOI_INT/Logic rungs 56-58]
   // When program control is 1 and the command echo is the C2 cal command #102, the command echo and status are copied to the Status_Return and Cmd Status tags.  This is for reference if the user wishes to reference the status later.
   56: EQU(C2_cal_ctrl,1)EQU(Inp_hi1769.CommandEcho,102)[COP(Inp_hi1769.CommandEcho,Status_Return,1) ,COP(Inp_hi1769.CommandStatus,cmd_status,1) ,MOV(2,C2_cal_ctrl) ];
   // Once the command is completed, this timer starts that will give enough delay before clearing the command so the status on the HMI will remain long enough for the user to see.
   57: EQU(C2_cal_ctrl,2)[TON(C2_cmd_reset_timer,?,?) ,XIC(C2_cmd_reset_timer.DN) MOV(3,C2_cal_ctrl) ];
   // Once the delay timer has run out, this rung will reset the status and clear the command.
   // The ctrl register is also reset.
   58: EQU(C2_cal_ctrl,3)[MOV(100,cmd_status) ,CLR(Out_hi1769.Command) ,OTU(C2_cal_cmd) ,MOV(0,C2_cal_ctrl) ];
